FUNCTION "CENTR. 1  ANTERIORE DX" : VOID
TITLE =CENTRATORE ANTERIORE DX
VERSION : 0.1

BEGIN
NETWORK
TITLE =LETTURA STATUS WORD DA DRIVE
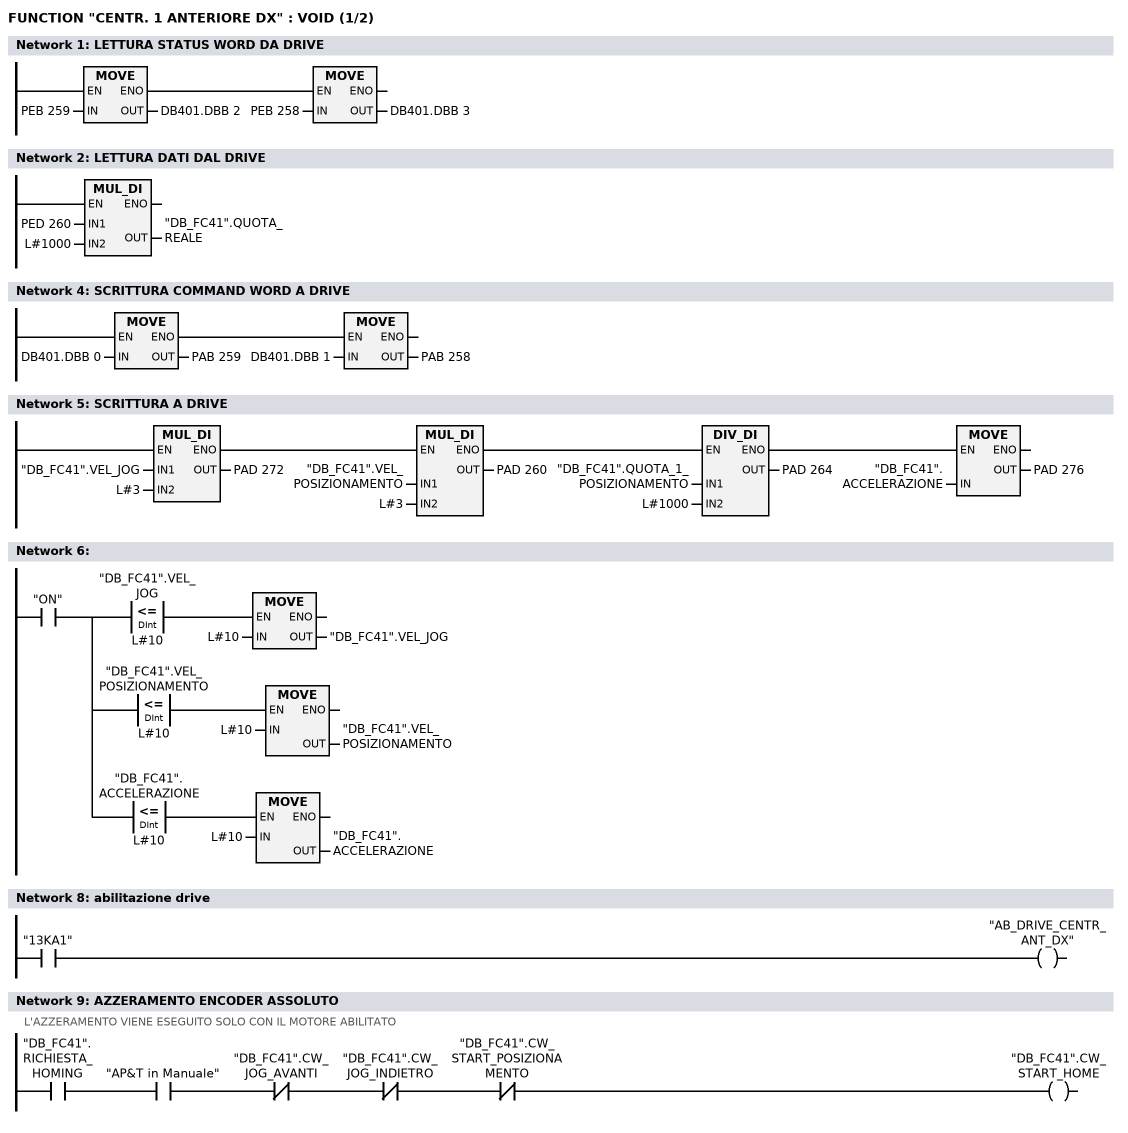
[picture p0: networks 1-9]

      U(    ;
      L     PEB  259;
      T     DB401.DBB    2;
      SET   ;
      SAVE  ;
      CLR   ;
      U     BIE;
      )     ;
      SPBNB _001;
      L     PEB  258;
      T     DB401.DBB    3;
_001: NOP   0;
NETWORK
TITLE =LETTURA DATI DAL DRIVE

      L     PED  260;
      L     L#1000;
      *D    ;
      T     "DB_FC41".QUOTA_REALE;
      NOP   0;
NETWORK
TITLE =

NETWORK
TITLE =SCRITTURA COMMAND WORD A DRIVE

      U(    ;
      L     DB401.DBB    0;
      T     PAB  259;
      SET   ;
      SAVE  ;
      CLR   ;
      U     BIE;
      )     ;
      SPBNB _002;
      L     DB401.DBB    1;
      T     PAB  258;
_002: NOP   0;
NETWORK
TITLE =SCRITTURA A DRIVE

      U(    ;
      U(    ;
      U(    ;
      L     "DB_FC41".VEL_JOG;
      L     L#3;
      *D    ;
      T     PAD  272;
      UN    OV;
      SAVE  ;
      CLR   ;
      U     BIE;
      )     ;
      SPBNB _003;
      L     "DB_FC41".VEL_POSIZIONAMENTO;
      L     L#3;
      *D    ;
      T     PAD  260;
      UN    OV;
      SAVE  ;
      CLR   ;
_003: U     BIE;
      )     ;
      SPBNB _004;
      L     "DB_FC41".QUOTA_1_POSIZIONAMENTO;
      L     L#1000;
      /D    ;
      T     PAD  264;
      UN    OV;
      SAVE  ;
      CLR   ;
_004: U     BIE;
      )     ;
      SPBNB _005;
      L     "DB_FC41".ACCELERAZIONE;
      T     PAD  276;
_005: NOP   0;
NETWORK
TITLE =

      U     "ON";
      =     L      0.0;
      U     L      0.0;
      U(    ;
      L     "DB_FC41".VEL_JOG;
      L     L#10;
      <=D   ;
      )     ;
      SPBNB _006;
      L     L#10;
      T     "DB_FC41".VEL_JOG;
_006: NOP   0;
      U     L      0.0;
      U(    ;
      L     "DB_FC41".VEL_POSIZIONAMENTO;
      L     L#10;
      <=D   ;
      )     ;
      SPBNB _007;
      L     L#10;
      T     "DB_FC41".VEL_POSIZIONAMENTO;
_007: NOP   0;
      U     L      0.0;
      U(    ;
      L     "DB_FC41".ACCELERAZIONE;
      L     L#10;
      <=D   ;
      )     ;
      SPBNB _008;
      L     L#10;
      T     "DB_FC41".ACCELERAZIONE;
_008: NOP   0;
NETWORK
TITLE =

NETWORK
TITLE =abilitazione drive

      U     "13KA1";
      =     "AB_DRIVE_CENTR_ANT_DX";
NETWORK
TITLE =AZZERAMENTO ENCODER ASSOLUTO
//L'AZZERAMENTO VIENE ESEGUITO SOLO CON IL MOTORE ABILITATO
      U     "DB_FC41".RICHIESTA_HOMING;
      U     "AP&T in Manuale";
      UN    "DB_FC41".CW_JOG_AVANTI;
      UN    "DB_FC41".CW_JOG_INDIETRO;
      UN    "DB_FC41".CW_START_POSIZIONAMENTO;
      =     "DB_FC41".CW_START_HOME;
NETWORK
TITLE =COMANDI DI JOG
//N.B. VERIFICARE QUOTE EXTRACORSA SOFTWARE
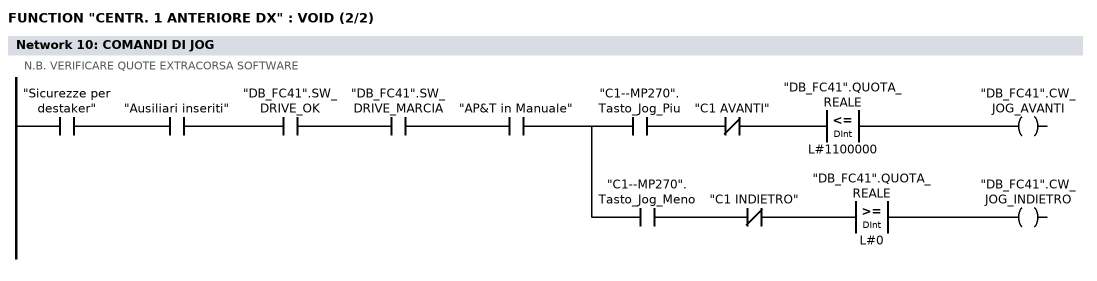
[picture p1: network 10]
      U     "Sicurezze per destaker";
      U     "Ausiliari inseriti";
      U     "DB_FC41".SW_DRIVE_OK;
      U     "DB_FC41".SW_DRIVE_MARCIA;
      U     "AP&T in Manuale";
      =     L      0.0;
      U     L      0.0;
      U     "C1--MP270".Tasto_Jog_Piu;
      UN    "C1 AVANTI";
      U(    ;
      L     "DB_FC41".QUOTA_REALE;
      L     L#1100000;
      <=D   ;
      )     ;
      =     "DB_FC41".CW_JOG_AVANTI;
      U     L      0.0;
      U     "C1--MP270".Tasto_Jog_Meno;
      UN    "C1 INDIETRO";
      U(    ;
      L     "DB_FC41".QUOTA_REALE;
      L     L#0;
      >=D   ;
      )     ;
      =     "DB_FC41".CW_JOG_INDIETRO;
NETWORK
TITLE =Centratore 1: Posizioni
//N.B. VERIFICARE QUOTE DI CONTROLLO
      U     "ON";
      =     L      0.0;
      U     L      0.0;
      U(    ;
      L     "DB_FC41".QUOTA_REALE;
      L     L#100;
      <=D   ;
      )     ;
      U(    ;
      L     "DB_FC41".QUOTA_REALE;
      L     L#-100;
      >=D   ;
      )     ;
      =     "C1: Asse in pos.0";
      U(    ;
      U(    ;
      U     L      0.0;
      SPBNB _009;
      L     "MATRICOLA ATTUALE".C1_Posizione_1;
      L     L#100;
      -D    ;
      T     "CONFRONTI CENTRATORI".C1_Pos_1_Min;
      UN    OV;
      SAVE  ;
      CLR   ;
_009: U     BIE;
      )     ;
      SPBNB _00a;
      L     "MATRICOLA ATTUALE".C1_Posizione_1;
      L     L#200;
      +D    ;
      T     "CONFRONTI CENTRATORI".C1_Pos_1_Max;
      UN    OV;
      SAVE  ;
      CLR   ;
_00a: U     BIE;
      )     ;
      U(    ;
      L     "DB_FC41".QUOTA_REALE;
      L     "CONFRONTI CENTRATORI".C1_Pos_1_Min;
      >=D   ;
      )     ;
      U(    ;
      L     "DB_FC41".QUOTA_REALE;
      L     "CONFRONTI CENTRATORI".C1_Pos_1_Max;
      <=D   ;
      )     ;
      =     "C1: Asse in pos.1";
      U(    ;
      U(    ;
      U     L      0.0;
      SPBNB _00b;
      L     "MATRICOLA ATTUALE".C1_Posizione_2;
      L     L#100;
      -D    ;
      T     "CONFRONTI CENTRATORI".C1_Pos_2_Min;
      UN    OV;
      SAVE  ;
      CLR   ;
_00b: U     BIE;
      )     ;
      SPBNB _00c;
      L     "MATRICOLA ATTUALE".C1_Posizione_2;
      L     L#50000;
      +D    ;
      T     "CONFRONTI CENTRATORI".C1_Pos_2_Max;
      UN    OV;
      SAVE  ;
      CLR   ;
_00c: U     BIE;
      )     ;
      U(    ;
      L     "DB_FC41".QUOTA_REALE;
      L     "CONFRONTI CENTRATORI".C1_Pos_2_Min;
      >=D   ;
      )     ;
      UN    "C1: Asse in pos.3";
      UN    "C1: Asse in pos.4";
      =     "C1: Asse in pos.2";
      U(    ;
      U(    ;
      U     L      0.0;
      SPBNB _00d;
      L     "MATRICOLA ATTUALE".C1_Posizione_3;
      L     L#100;
      -D    ;
      T     "CONFRONTI CENTRATORI".C1_Pos_3_Min;
      UN    OV;
      SAVE  ;
      CLR   ;
_00d: U     BIE;
      )     ;
      SPBNB _00e;
      L     "MATRICOLA ATTUALE".C1_Posizione_3;
      L     L#50000;
      +D    ;
      T     "CONFRONTI CENTRATORI".C1_Pos_3_Max;
      UN    OV;
      SAVE  ;
      CLR   ;
_00e: U     BIE;
      )     ;
      U(    ;
      L     "DB_FC41".QUOTA_REALE;
      L     "CONFRONTI CENTRATORI".C1_Pos_3_Min;
      >=D   ;
      )     ;
      UN    "C1: Asse in pos.4";
      =     "C1: Asse in pos.3";
      U(    ;
      U(    ;
      U     L      0.0;
      SPBNB _00f;
      L     "MATRICOLA ATTUALE".C1_Posizione_4;
      L     L#100;
      -D    ;
      T     "CONFRONTI CENTRATORI".C1_Pos_4_Min;
      UN    OV;
      SAVE  ;
      CLR   ;
_00f: U     BIE;
      )     ;
      SPBNB _010;
      L     "MATRICOLA ATTUALE".C1_Posizione_4;
      L     L#100;
      +D    ;
      T     "CONFRONTI CENTRATORI".C1_Pos_4_Max;
      UN    OV;
      SAVE  ;
      CLR   ;
_010: U     BIE;
      )     ;
      U(    ;
      L     "DB_FC41".QUOTA_REALE;
      L     "CONFRONTI CENTRATORI".C1_Pos_4_Min;
      >=D   ;
      )     ;
      U(    ;
      L     "DB_FC41".QUOTA_REALE;
      L     "CONFRONTI CENTRATORI".C1_Pos_4_Max;
      <=D   ;
      )     ;
      =     "C1: Asse in pos.4";
NETWORK
TITLE =Centratore 1: consenso abilitazione passi
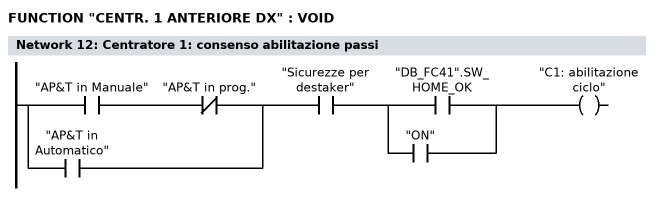
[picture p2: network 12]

      U(    ;
      U     "AP&T in Manuale";
      UN    "AP&T in prog.";
      O     "AP&T in Automatico";
      )     ;
      U     "Sicurezze per destaker";
      U(    ;
      O     "DB_FC41".SW_HOME_OK;
      O     "ON";
      )     ;
      =     "C1: abilitazione ciclo";
NETWORK
TITLE =Centratore 1: comando avvicinamento  (centraggi aperti)

      U(    ;
      U(    ;
      O     "Comando apre centraggi";
      O     "C1--MP270".Tasto_Indietro;
      O     ;
      U     "Apertura centratori";
      U(    ;
      O     "Centratori a riposo";
      O     "Centratori tutti chiusi";
      )     ;
      )     ;
      UN    "C1: Asse in pos.1";
      UN    "C1: comando arrivo";
      UN    "C1: comando a riposo";
      U     "C1: abilitazione ciclo";
      L     S5T#100MS;
      SE    T    180;
      NOP   0;
      NOP   0;
      NOP   0;
      U     T    180;
      )     ;
      S     "C1: comando avvicinam";
      U(    ;
      O     "C1: Asse in pos.1";
      O(    ;
      U(    ;
      O     "Ripristino centratori";
      O     "Comando riposo centraggi";
      O     "C1--MP270".Tasto_Riposo;
      )     ;
      FP    "C1: one shot 1";
      )     ;
      )     ;
      R     "C1: comando avvicinam";
      NOP   0;
NETWORK
TITLE =Centratore 1: comando arrivo (centraggi chiusi)

      U(    ;
      U(    ;
      O     "Comando chiude centraggi";
      O     "C1--MP270".Tasto_Avanti;
      O     ;
      U     "Chiusura centratori";
      U(    ;
      O     "Centratori tutti aperti";
      O     "Centratori a riposo";
      )     ;
      )     ;
      UN    "C1: Asse in pos.4";
      UN    "C1: comando avvicinam";
      UN    "C1: comando a riposo";
      U     "C1: abilitazione ciclo";
      L     S5T#100MS;
      SE    T    181;
      NOP   0;
      NOP   0;
      NOP   0;
      U     T    181;
      )     ;
      S     "C1: comando arrivo";
      U(    ;
      O     "C1: Asse in pos.4";
      O(    ;
      U(    ;
      O     "Ripristino centratori";
      O     "Comando riposo centraggi";
      O     "C1--MP270".Tasto_Riposo;
      )     ;
      FP    "C1: one shot 2";
      )     ;
      )     ;
      R     "C1: comando arrivo";
      NOP   0;
NETWORK
TITLE =Centratore 1: comando automatico centraggi a riposo

      U(    ;
      U(    ;
      O     "Comando riposo centraggi";
      O     "C1--MP270".Tasto_Riposo;
      )     ;
      UN    "C1: Asse in pos.0";
      UN    "C1: comando avvicinam";
      UN    "C1: comando arrivo";
      U     "C1: abilitazione ciclo";
      L     S5T#100MS;
      SE    T    182;
      NOP   0;
      NOP   0;
      NOP   0;
      U     T    182;
      )     ;
      S     "C1: comando a riposo";
      U(    ;
      O     "C1: Asse in pos.0";
      O(    ;
      U     "Ripristino centratori";
      FP    "C1: one shot 3";
      )     ;
      )     ;
      R     "C1: comando a riposo";
      NOP   0;
NETWORK
TITLE =Centratore 1: quote impostate per posizioni

      U     "ON";
      =     L      0.0;
      U(    ;
      U(    ;
      U     L      0.0;
      U     "C1: comando a riposo";
      UN    "C1: Asse in pos.0";
      SPBNB _011;
      L     0;
      T     "DB_FC41".QUOTA_1_POSIZIONAMENTO;
      SET   ;
      SAVE  ;
      CLR   ;
_011: U     BIE;
      )     ;
      SPBNB _012;
      L     L#150;
      T     "DB_FC41".VEL_POSIZIONAMENTO;
      SET   ;
      SAVE  ;
      CLR   ;
_012: U     BIE;
      )     ;
      SPBNB _013;
      L     L#1000;
      T     "DB_FC41".ACCELERAZIONE;
      SET   ;
      SAVE  ;
      CLR   ;
_013: U     BIE;
      =     "C1: Quote pronte pos.0";
      U(    ;
      U(    ;
      U     L      0.0;
      U     "C1: comando avvicinam";
      UN    "C1: Asse in pos.1";
      SPBNB _014;
      L     "MATRICOLA ATTUALE".C1_Posizione_1;
      T     "DB_FC41".QUOTA_1_POSIZIONAMENTO;
      SET   ;
      SAVE  ;
      CLR   ;
_014: U     BIE;
      )     ;
      SPBNB _015;
      L     "MATRICOLA ATTUALE".C1_Velocita_1;
      T     "DB_FC41".VEL_POSIZIONAMENTO;
      SET   ;
      SAVE  ;
      CLR   ;
_015: U     BIE;
      )     ;
      SPBNB _016;
      L     "MATRICOLA ATTUALE".C1_Accell_1;
      T     "DB_FC41".ACCELERAZIONE;
      SET   ;
      SAVE  ;
      CLR   ;
_016: U     BIE;
      =     "C1: Quote pronte pos.1";
      U     L      0.0;
      U     "C1: comando arrivo";
      =     L      0.1;
      U(    ;
      U(    ;
      U     L      0.1;
      UN    "C1: Asse in pos.2";
      SPBNB _017;
      L     "MATRICOLA ATTUALE".C1_Posizione_4;
      T     "DB_FC41".QUOTA_1_POSIZIONAMENTO;
      SET   ;
      SAVE  ;
      CLR   ;
_017: U     BIE;
      )     ;
      SPBNB _018;
      L     "MATRICOLA ATTUALE".C1_Velocita_2;
      T     "DB_FC41".VEL_POSIZIONAMENTO;
      SET   ;
      SAVE  ;
      CLR   ;
_018: U     BIE;
      )     ;
      SPBNB _019;
      L     "MATRICOLA ATTUALE".C1_Accell_2;
      T     "DB_FC41".ACCELERAZIONE;
      SET   ;
      SAVE  ;
      CLR   ;
_019: U     BIE;
      S     "C1: Quote pronte pos.2";
      U     L      0.1;
      U     "C1: Quote pronte pos.2";
      UN    "C1: Reset start pos.2";
      L     S5T#1S;
      SE    "C1: ritardo P2";
      NOP   0;
      NOP   0;
      NOP   0;
      U     "C1: ritardo P2";
      S     "C1: Reset start pos.2";
      R     "C1: Quote pronte pos.2";
      U     L      0.0;
      U     "C1: comando arrivo";
      =     L      0.1;
      U(    ;
      U(    ;
      U(    ;
      U     L      0.1;
      U     "C1: Asse in pos.2";
      UN    "C1: Asse in pos.3";
      SPBNB _01a;
      L     "MATRICOLA ATTUALE".C1_Posizione_4;
      T     "DB_FC41".VEL_POSIZIONAMENTO;
      SET   ;
      SAVE  ;
      CLR   ;
_01a: U     BIE;
      )     ;
      SPBNB _01b;
      L     "MATRICOLA ATTUALE".C1_Velocita_3;
      T     "DB_FC41".VEL_POSIZIONAMENTO;
      SET   ;
      SAVE  ;
      CLR   ;
_01b: U     BIE;
      )     ;
      SPBNB _01c;
      L     "MATRICOLA ATTUALE".C1_Accell_3;
      T     "DB_FC41".ACCELERAZIONE;
      SET   ;
      SAVE  ;
      CLR   ;
_01c: U     BIE;
      )     ;
      U     "C1: Reset start pos.2";
      S     "C1: Quote pronte pos.3";
      R     "C1: Reset start pos.2";
      U     L      0.1;
      U     "C1: Quote pronte pos.3";
      L     S5T#500MS;
      SE    "C1: ritardo P3";
      NOP   0;
      NOP   0;
      NOP   0;
      U     "C1: ritardo P3";
      S     "C1: Reset start pos.3";
      R     "C1: Quote pronte pos.3";
      U     L      0.0;
      U     "C1: comando arrivo";
      =     L      0.1;
      U(    ;
      U(    ;
      U(    ;
      U     L      0.1;
      U     "C1: Asse in pos.3";
      UN    "C1: Asse in pos.4";
      SPBNB _01d;
      L     "MATRICOLA ATTUALE".C1_Posizione_4;
      T     "DB_FC41".VEL_POSIZIONAMENTO;
      SET   ;
      SAVE  ;
      CLR   ;
_01d: U     BIE;
      )     ;
      SPBNB _01e;
      L     "MATRICOLA ATTUALE".C1_Velocita_4;
      T     "DB_FC41".VEL_POSIZIONAMENTO;
      SET   ;
      SAVE  ;
      CLR   ;
_01e: U     BIE;
      )     ;
      SPBNB _01f;
      L     "MATRICOLA ATTUALE".C1_Accell_4;
      T     "DB_FC41".ACCELERAZIONE;
      SET   ;
      SAVE  ;
      CLR   ;
_01f: U     BIE;
      )     ;
      U     "C1: Reset start pos.3";
      S     "C1: Quote pronte pos.4";
      R     "C1: Reset start pos.3";
      U     L      0.1;
      U     "C1: Quote pronte pos.4";
      L     S5T#500MS;
      SE    "C1: ritardo P4";
      NOP   0;
      NOP   0;
      NOP   0;
      U     "C1: ritardo P4";
      S     "C1: Reset start pos.4";
      R     "C1: Quote pronte pos.4";
NETWORK
TITLE =Centratore 1: reset impostate
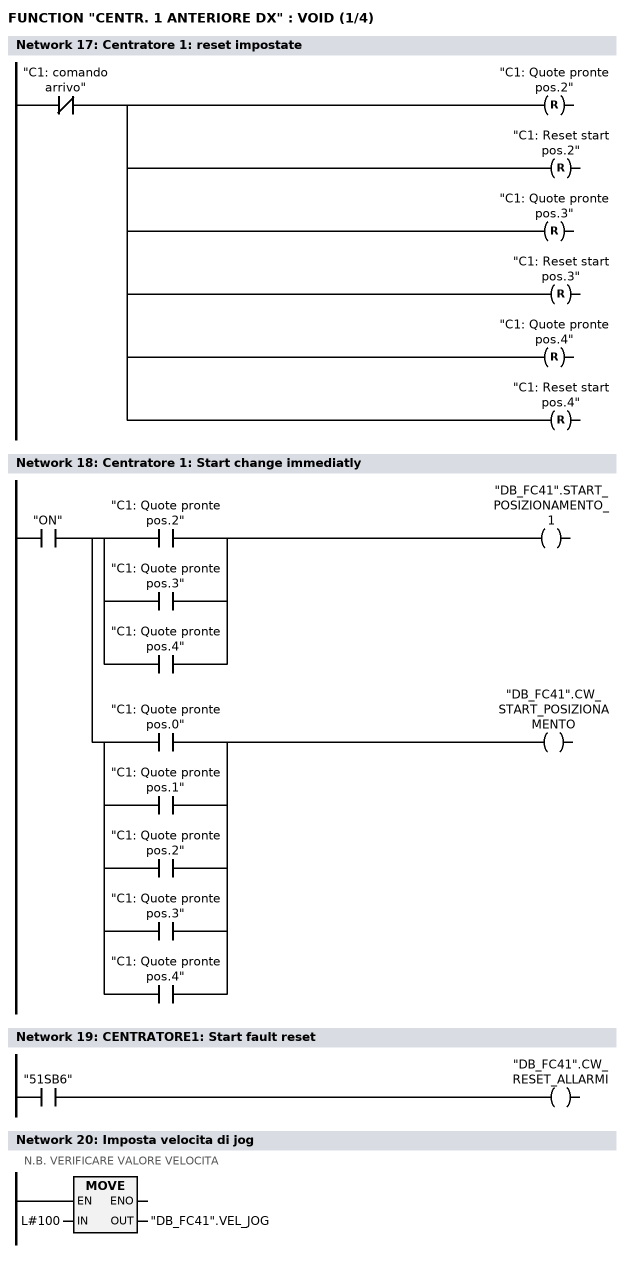
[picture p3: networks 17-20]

      UN    "C1: comando arrivo";
      R     "C1: Quote pronte pos.2";
      R     "C1: Reset start pos.2";
      R     "C1: Quote pronte pos.3";
      R     "C1: Reset start pos.3";
      R     "C1: Quote pronte pos.4";
      R     "C1: Reset start pos.4";
NETWORK
TITLE =Centratore 1: Start change immediatly

      U     "ON";
      =     L      0.0;
      U     L      0.0;
      U(    ;
      O     "C1: Quote pronte pos.2";
      O     "C1: Quote pronte pos.3";
      O     "C1: Quote pronte pos.4";
      )     ;
      =     "DB_FC41".START_POSIZIONAMENTO_1;
      U     L      0.0;
      U(    ;
      O     "C1: Quote pronte pos.0";
      O     "C1: Quote pronte pos.1";
      O     "C1: Quote pronte pos.2";
      O     "C1: Quote pronte pos.3";
      O     "C1: Quote pronte pos.4";
      )     ;
      =     "DB_FC41".CW_START_POSIZIONAMENTO;
NETWORK
TITLE =CENTRATORE1: Start fault reset

      U     "51SB6";
      =     "DB_FC41".CW_RESET_ALLARMI;
NETWORK
TITLE =Imposta velocita di jog
//N.B. VERIFICARE VALORE VELOCITA
      L     L#100;
      T     "DB_FC41".VEL_JOG;
      NOP   0;
NETWORK
TITLE =Centratore 1: Drive Enable ok
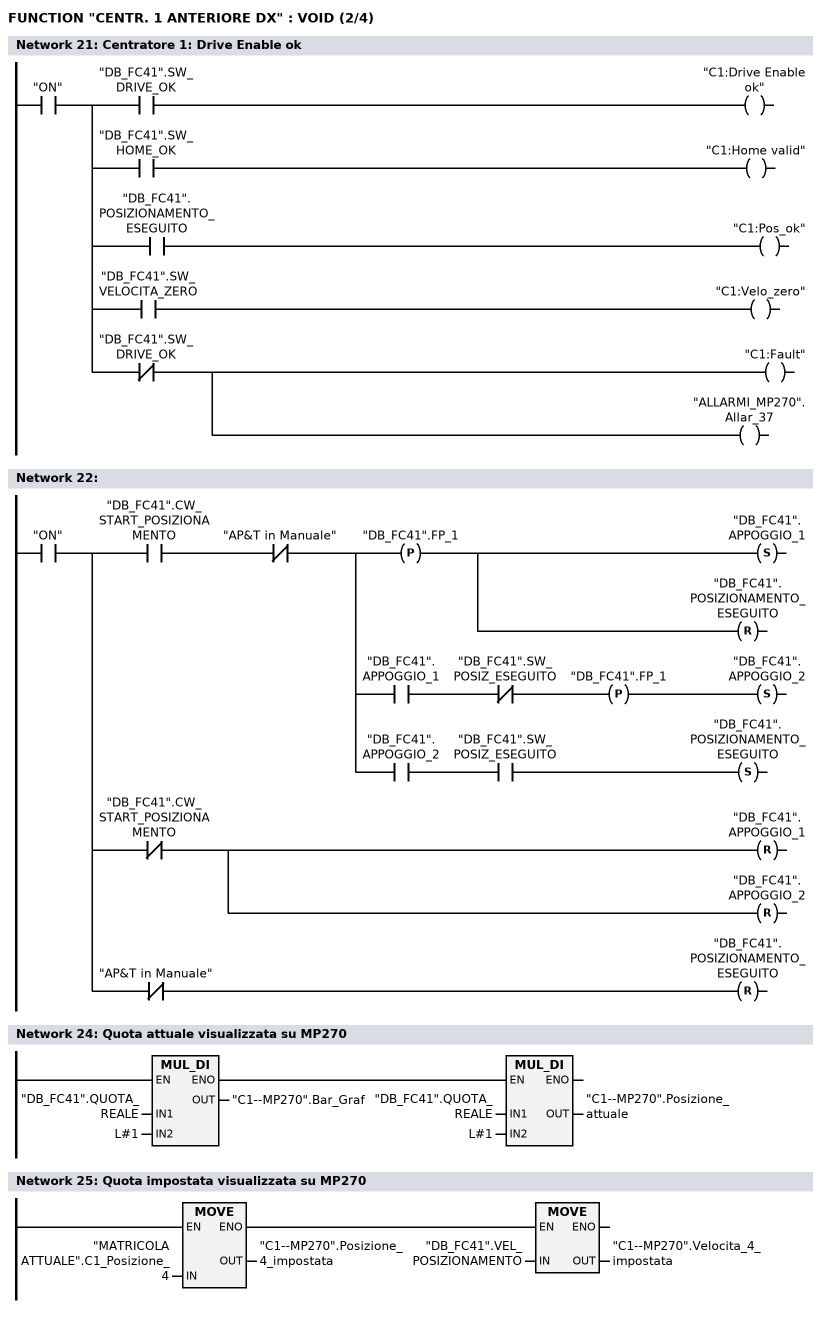
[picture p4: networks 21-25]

      U     "ON";
      =     L      0.0;
      U     L      0.0;
      U     "DB_FC41".SW_DRIVE_OK;
      =     "C1:Drive Enable ok";
      U     L      0.0;
      U     "DB_FC41".SW_HOME_OK;
      =     "C1:Home valid";
      U     L      0.0;
      U     "DB_FC41".POSIZIONAMENTO_ESEGUITO;
      =     "C1:Pos_ok";
      U     L      0.0;
      U     "DB_FC41".SW_VELOCITA_ZERO;
      =     "C1:Velo_zero";
      U     L      0.0;
      UN    "DB_FC41".SW_DRIVE_OK;
      =     "C1:Fault";
      =     "ALLARMI_MP270".Allar_37;
NETWORK
TITLE =

      U     "ON";
      =     L      0.0;
      U     L      0.0;
      U     "DB_FC41".CW_START_POSIZIONAMENTO;
      UN    "AP&T in Manuale";
      =     L      0.1;
      U     L      0.1;
      FP    "DB_FC41".FP_1;
      S     "DB_FC41".APPOGGIO_1;
      R     "DB_FC41".POSIZIONAMENTO_ESEGUITO;
      U     L      0.1;
      U     "DB_FC41".APPOGGIO_1;
      UN    "DB_FC41".SW_POSIZ_ESEGUITO;
      FP    "DB_FC41".FP_1;
      S     "DB_FC41".APPOGGIO_2;
      U     L      0.1;
      U     "DB_FC41".APPOGGIO_2;
      U     "DB_FC41".SW_POSIZ_ESEGUITO;
      S     "DB_FC41".POSIZIONAMENTO_ESEGUITO;
      U     L      0.0;
      UN    "DB_FC41".CW_START_POSIZIONAMENTO;
      R     "DB_FC41".APPOGGIO_1;
      R     "DB_FC41".APPOGGIO_2;
      U     L      0.0;
      UN    "AP&T in Manuale";
      R     "DB_FC41".POSIZIONAMENTO_ESEGUITO;
NETWORK
TITLE =

NETWORK
TITLE =Quota attuale visualizzata su MP270

      U(    ;
      L     "DB_FC41".QUOTA_REALE;
      L     L#1;
      *D    ;
      T     "C1--MP270".Bar_Graf;
      UN    OV;
      SAVE  ;
      CLR   ;
      U     BIE;
      )     ;
      SPBNB _020;
      L     "DB_FC41".QUOTA_REALE;
      L     L#1;
      *D    ;
      T     "C1--MP270".Posizione_attuale;
_020: NOP   0;
NETWORK
TITLE =Quota impostata visualizzata su MP270

      U(    ;
      L     "MATRICOLA ATTUALE".C1_Posizione_4;
      T     "C1--MP270".Posizione_4_impostata;
      SET   ;
      SAVE  ;
      CLR   ;
      U     BIE;
      )     ;
      SPBNB _021;
      L     "DB_FC41".VEL_POSIZIONAMENTO;
      T     "C1--MP270".Velocita_4_impostata;
_021: NOP   0;
NETWORK
TITLE =Visualizza FC su MP270
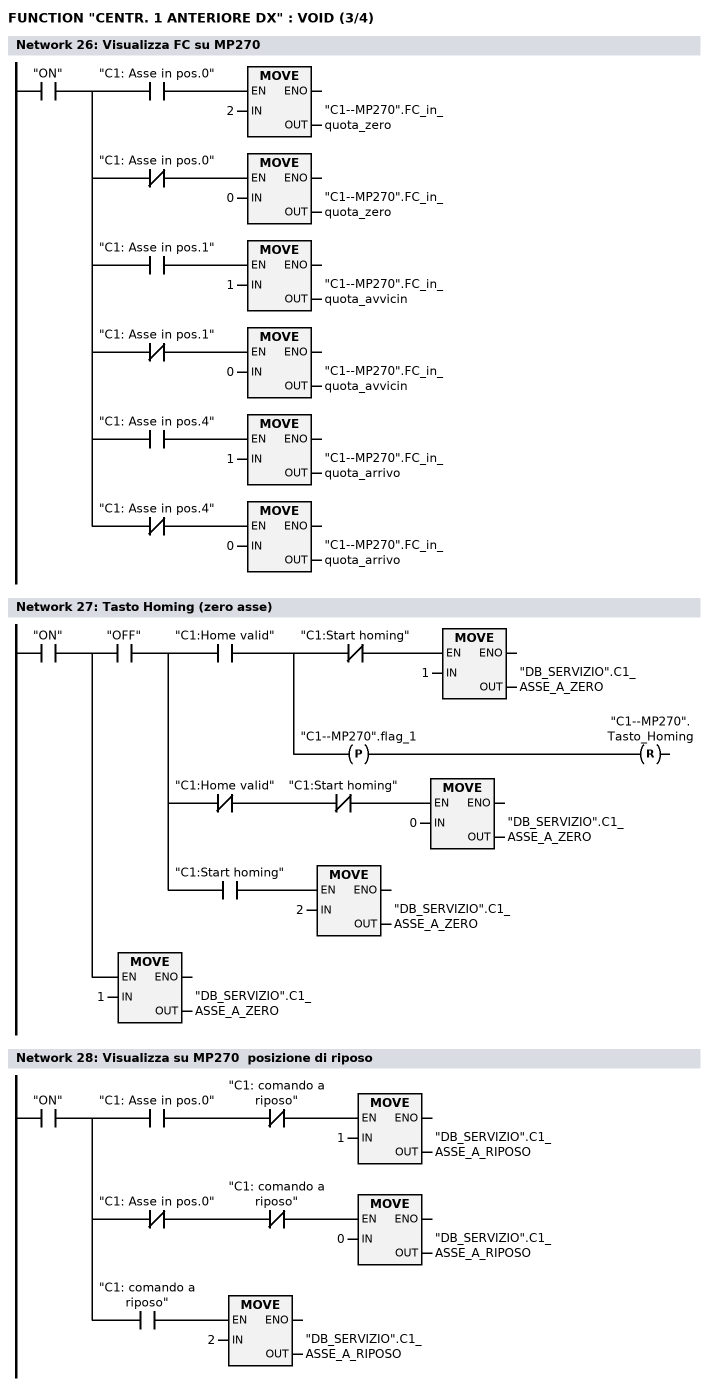
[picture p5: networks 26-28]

      U     "ON";
      =     L      0.0;
      U     L      0.0;
      U     "C1: Asse in pos.0";
      SPBNB _022;
      L     2;
      T     "C1--MP270".FC_in_quota_zero;
_022: NOP   0;
      U     L      0.0;
      UN    "C1: Asse in pos.0";
      SPBNB _023;
      L     0;
      T     "C1--MP270".FC_in_quota_zero;
_023: NOP   0;
      U     L      0.0;
      U     "C1: Asse in pos.1";
      SPBNB _024;
      L     1;
      T     "C1--MP270".FC_in_quota_avvicin;
_024: NOP   0;
      U     L      0.0;
      UN    "C1: Asse in pos.1";
      SPBNB _025;
      L     0;
      T     "C1--MP270".FC_in_quota_avvicin;
_025: NOP   0;
      U     L      0.0;
      U     "C1: Asse in pos.4";
      SPBNB _026;
      L     1;
      T     "C1--MP270".FC_in_quota_arrivo;
_026: NOP   0;
      U     L      0.0;
      UN    "C1: Asse in pos.4";
      SPBNB _027;
      L     0;
      T     "C1--MP270".FC_in_quota_arrivo;
_027: NOP   0;
NETWORK
TITLE =Tasto Homing (zero asse)

      U     "ON";
      =     L      0.0;
      U     L      0.0;
      U     "OFF";
      =     L      0.1;
      U     L      0.1;
      U     "C1:Home valid";
      =     L      0.2;
      U     L      0.2;
      UN    "C1:Start homing";
      SPBNB _028;
      L     1;
      T     "DB_SERVIZIO".C1_ASSE_A_ZERO;
_028: NOP   0;
      U     L      0.2;
      FP    "C1--MP270".flag_1;
      R     "C1--MP270".Tasto_Homing;
      U     L      0.1;
      UN    "C1:Home valid";
      UN    "C1:Start homing";
      SPBNB _029;
      L     0;
      T     "DB_SERVIZIO".C1_ASSE_A_ZERO;
_029: NOP   0;
      U     L      0.1;
      U     "C1:Start homing";
      SPBNB _02a;
      L     2;
      T     "DB_SERVIZIO".C1_ASSE_A_ZERO;
_02a: NOP   0;
      U     L      0.0;
      SPBNB _02b;
      L     1;
      T     "DB_SERVIZIO".C1_ASSE_A_ZERO;
_02b: NOP   0;
NETWORK
TITLE =Visualizza su MP270  posizione di riposo

      U     "ON";
      =     L      0.0;
      U     L      0.0;
      U     "C1: Asse in pos.0";
      UN    "C1: comando a riposo";
      SPBNB _02c;
      L     1;
      T     "DB_SERVIZIO".C1_ASSE_A_RIPOSO;
_02c: NOP   0;
      U     L      0.0;
      UN    "C1: Asse in pos.0";
      UN    "C1: comando a riposo";
      SPBNB _02d;
      L     0;
      T     "DB_SERVIZIO".C1_ASSE_A_RIPOSO;
_02d: NOP   0;
      U     L      0.0;
      U     "C1: comando a riposo";
      SPBNB _02e;
      L     2;
      T     "DB_SERVIZIO".C1_ASSE_A_RIPOSO;
_02e: NOP   0;
NETWORK
TITLE =Visualizza su MP270  posizione di avvicinamento
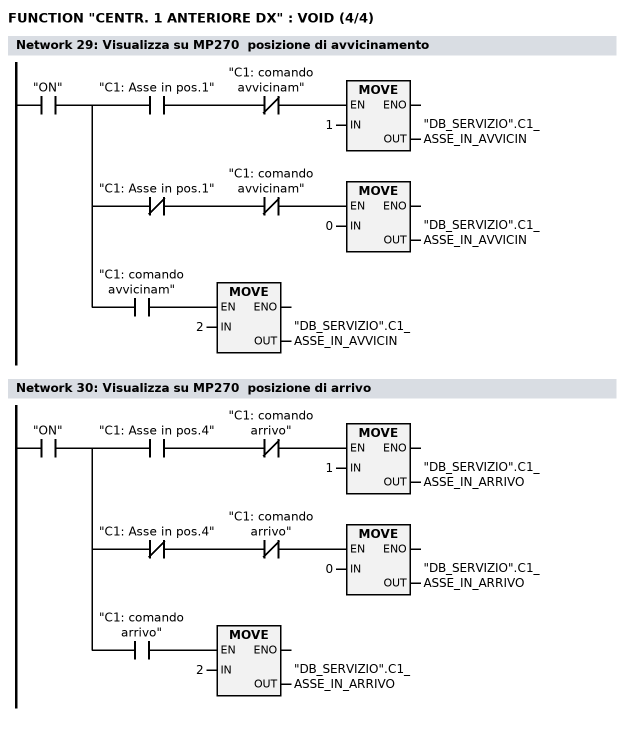
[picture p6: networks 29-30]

      U     "ON";
      =     L      0.0;
      U     L      0.0;
      U     "C1: Asse in pos.1";
      UN    "C1: comando avvicinam";
      SPBNB _02f;
      L     1;
      T     "DB_SERVIZIO".C1_ASSE_IN_AVVICIN;
_02f: NOP   0;
      U     L      0.0;
      UN    "C1: Asse in pos.1";
      UN    "C1: comando avvicinam";
      SPBNB _030;
      L     0;
      T     "DB_SERVIZIO".C1_ASSE_IN_AVVICIN;
_030: NOP   0;
      U     L      0.0;
      U     "C1: comando avvicinam";
      SPBNB _031;
      L     2;
      T     "DB_SERVIZIO".C1_ASSE_IN_AVVICIN;
_031: NOP   0;
NETWORK
TITLE =Visualizza su MP270  posizione di arrivo

      U     "ON";
      =     L      0.0;
      U     L      0.0;
      U     "C1: Asse in pos.4";
      UN    "C1: comando arrivo";
      SPBNB _032;
      L     1;
      T     "DB_SERVIZIO".C1_ASSE_IN_ARRIVO;
_032: NOP   0;
      U     L      0.0;
      UN    "C1: Asse in pos.4";
      UN    "C1: comando arrivo";
      SPBNB _033;
      L     0;
      T     "DB_SERVIZIO".C1_ASSE_IN_ARRIVO;
_033: NOP   0;
      U     L      0.0;
      U     "C1: comando arrivo";
      SPBNB _034;
      L     2;
      T     "DB_SERVIZIO".C1_ASSE_IN_ARRIVO;
_034: NOP   0;
END_FUNCTION

